(* Logix 5000 Routine export Unit1_EShutdown; software revision 20.05 *)

TYPE Unit_Type :   // Common information for a unit
STRUCT
   Alm_Reset : BOOL;   // Alarm reset
   Local : BOOL;   // Local/remote control indication
   Maint : BOOL;   // Maintenance privilege for device control
   Man_StartOpen : BOOL;   // Manual start/open from operator
   Man_StopClose : BOOL;   // Manual stop/close from operator
   Man_DevNum : DINT;   // Number of device started/stopped at OI
   Msg : DINT;   // Message number
   Time_Remaining : DINT;   // Remaining time in timed steps
END_STRUCT
END_TYPE

TYPE Seq_Type :   // Sequence Information
STRUCT
   Step_Num : DINT;   // Current step number
   Running : BOOL;   // Running indication
   PC_Start : BOOL;   // Sequence start request from PC
   LTP_Start : BOOL;   // Sequence start request from LTP
   Ons : BOOL;   // One-shot storage to start
   Auto_Start : BOOL;   // Auto-start request
   Auto_Ons : BOOL;   // Auto-start one-shot storage
   Req_Tmr : TIMER;   // Auto-start hold timer
END_STRUCT
END_TYPE

VAR_GLOBAL   (* controller tags *)
   Unit1_Hold : Seq_Type := (Req_Tmr.PRE := 5000);   // Unit Desc1 Hold Sequence
   Unit1_Sample : Seq_Type := (Req_Tmr.PRE := 5000);   // Unit Desc1 Sample Sequence
   Unit1_EShutdown_Tmr : TIMER := (PRE := 15000);   // Unit Desc1 E-Shutdown Timer
   Unit1 : Unit_Type;   // Unit Desc1
   Unit1_Shutdown : Seq_Type := (Req_Tmr.PRE := 5000);   // Unit Desc1 Shutdown Sequence
   Unit1_Eshutdown : Seq_Type := (Req_Tmr.PRE := 5000);   // Unit Desc1 E-Shutdown Sequence
END_VAR

PROGRAM MainProgram

ROUTINE Unit1_EShutdown   (* ladder *)
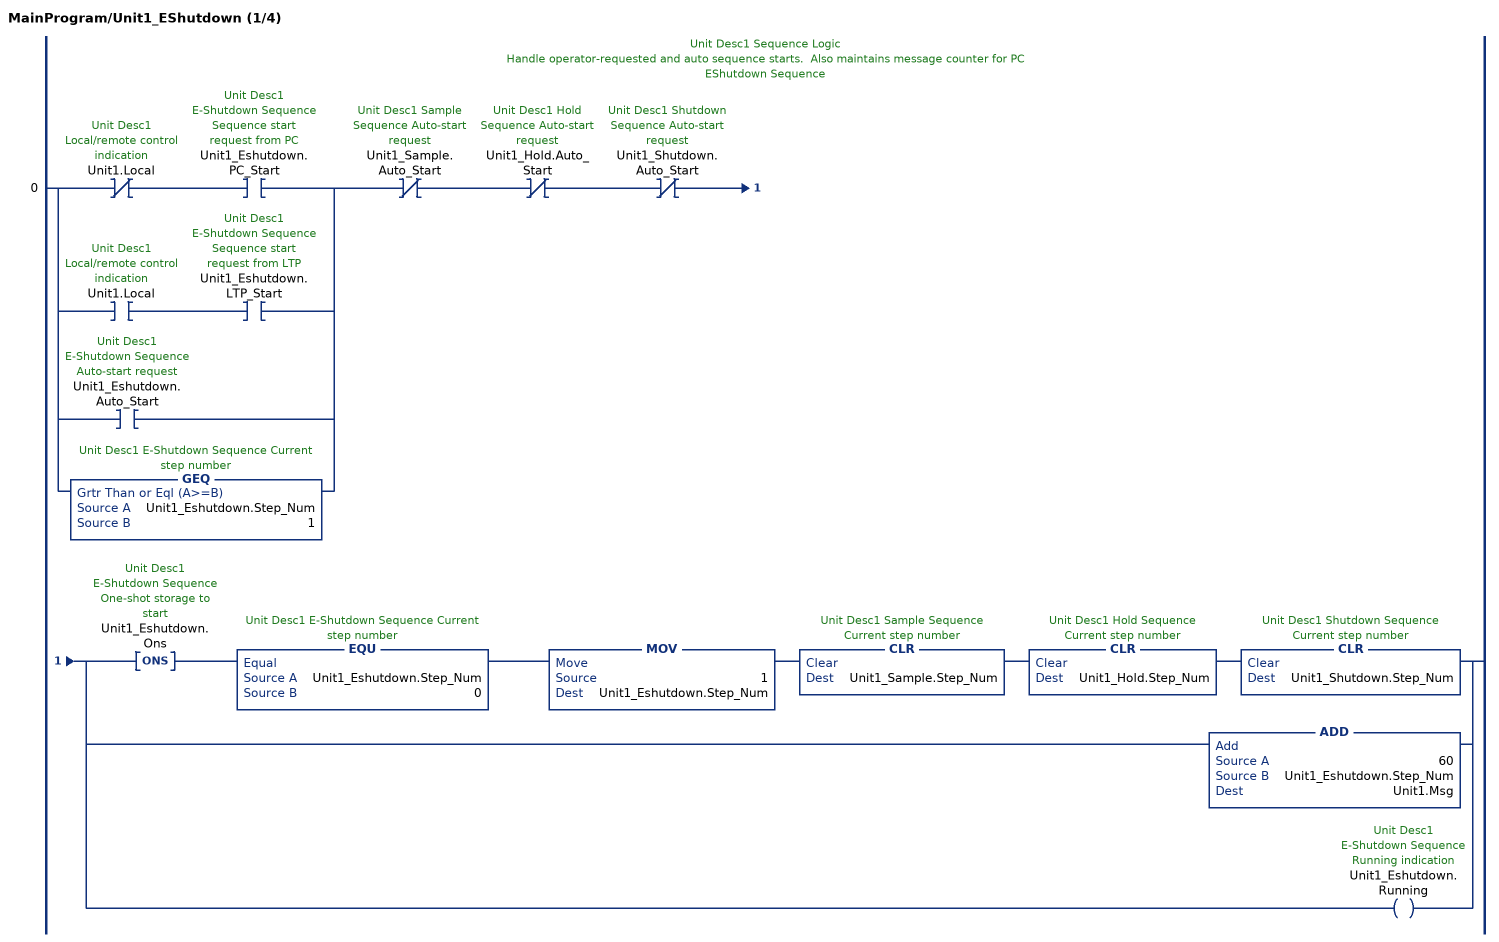
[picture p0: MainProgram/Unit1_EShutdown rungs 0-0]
   // Unit Desc1 Sequence Logic
   // Handle operator-requested and auto sequence starts.  Also maintains message counter for PC
   // EShutdown Sequence
   0: [XIO(Unit1.Local) XIC(Unit1_Eshutdown.PC_Start) ,XIC(Unit1.Local) XIC(Unit1_Eshutdown.LTP_Start) ,XIC(Unit1_Eshutdown.Auto_Start) ,GEQ(Unit1_Eshutdown.Step_Num,1) ]XIO(Unit1_Sample.Auto_Start)XIO(Unit1_Hold.Auto_Start)XIO(Unit1_Shutdown.Auto_Start)[ONS(Unit1_Eshutdown.Ons) EQU(Unit1_Eshutdown.Step_Num,0) MOV(1,Unit1_Eshutdown.Step_Num) CLR(Unit1_Sample.Step_Num) CLR(Unit1_Hold.Step_Num) CLR(Unit1_Shutdown.Step_Num) ,ADD(60,Unit1_Eshutdown.Step_Num,Unit1.Msg) ,OTE(Unit1_Eshutdown.Running) ];
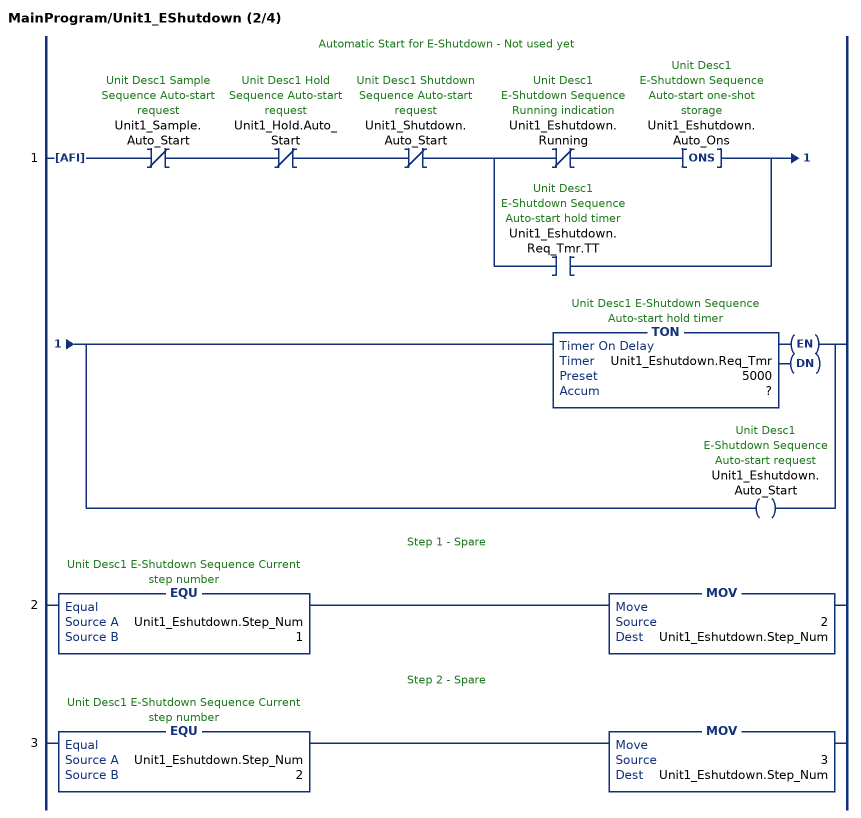
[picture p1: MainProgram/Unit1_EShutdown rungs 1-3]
   // Automatic Start for E-Shutdown - Not used yet
   1: AFI()XIO(Unit1_Sample.Auto_Start)XIO(Unit1_Hold.Auto_Start)XIO(Unit1_Shutdown.Auto_Start)[XIO(Unit1_Eshutdown.Running) ONS(Unit1_Eshutdown.Auto_Ons) ,XIC(Unit1_Eshutdown.Req_Tmr.TT) ][TON(Unit1_Eshutdown.Req_Tmr,?,?) ,OTE(Unit1_Eshutdown.Auto_Start) ];
   // Step 1 - Spare
   2: EQU(Unit1_Eshutdown.Step_Num,1)MOV(2,Unit1_Eshutdown.Step_Num);
   // Step 2 - Spare
   3: EQU(Unit1_Eshutdown.Step_Num,2)MOV(3,Unit1_Eshutdown.Step_Num);
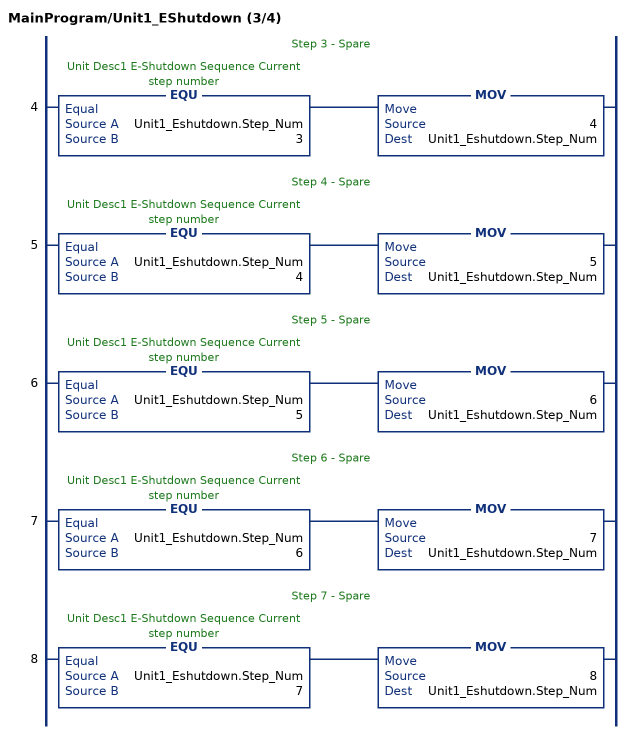
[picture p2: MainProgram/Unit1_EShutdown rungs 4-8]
   // Step 3 - Spare
   4: EQU(Unit1_Eshutdown.Step_Num,3)MOV(4,Unit1_Eshutdown.Step_Num);
   // Step 4 - Spare
   5: EQU(Unit1_Eshutdown.Step_Num,4)MOV(5,Unit1_Eshutdown.Step_Num);
   // Step 5 - Spare
   6: EQU(Unit1_Eshutdown.Step_Num,5)MOV(6,Unit1_Eshutdown.Step_Num);
   // Step 6 - Spare
   7: EQU(Unit1_Eshutdown.Step_Num,6)MOV(7,Unit1_Eshutdown.Step_Num);
   // Step 7 - Spare
   8: EQU(Unit1_Eshutdown.Step_Num,7)MOV(8,Unit1_Eshutdown.Step_Num);
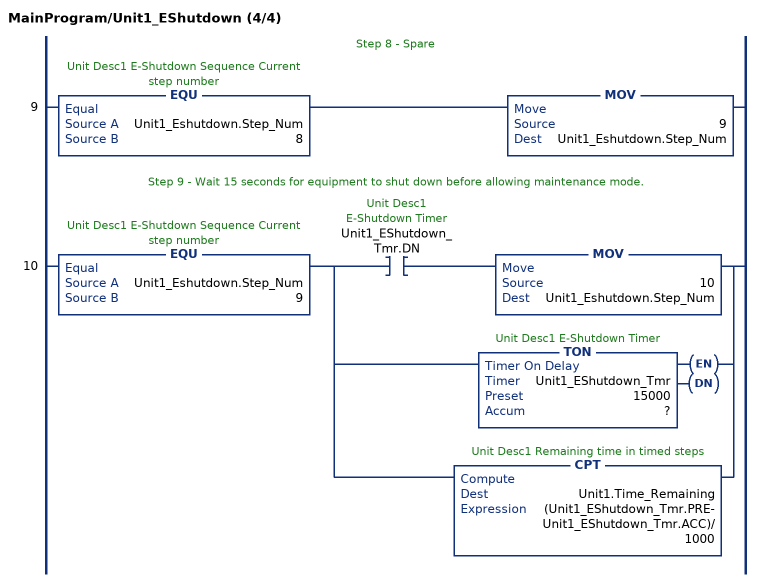
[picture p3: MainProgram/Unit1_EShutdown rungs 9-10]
   // Step 8 - Spare
   9: EQU(Unit1_Eshutdown.Step_Num,8)MOV(9,Unit1_Eshutdown.Step_Num);
   // Step 9 - Wait 15 seconds for equipment to shut down before allowing maintenance mode.
   10: EQU(Unit1_Eshutdown.Step_Num,9)[XIC(Unit1_EShutdown_Tmr.DN) MOV(10,Unit1_Eshutdown.Step_Num) ,TON(Unit1_EShutdown_Tmr,?,?) ,CPT(Unit1.Time_Remaining,(Unit1_EShutdown_Tmr.PRE-Unit1_EShutdown_Tmr.ACC)/1000) ];
END_ROUTINE
END_PROGRAM
